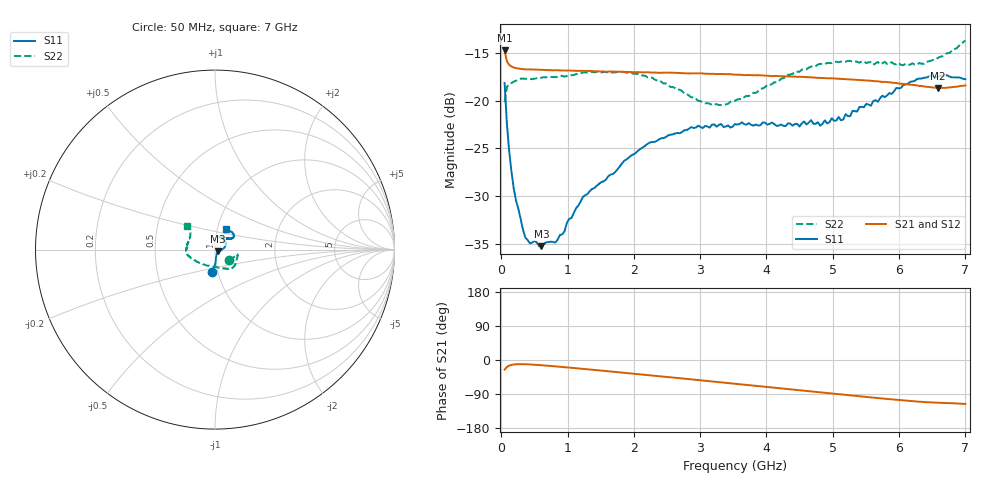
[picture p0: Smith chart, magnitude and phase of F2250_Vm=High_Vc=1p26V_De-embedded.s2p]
! Integrated Device Technology
! Corporate Headquarters
! 6024 Silver Creek Valley Road
! San Jose, CA 95138  USA
! Phone:  1-408-284-8200
! Toll Free:  1-800-223-1366
! Webpage:  http://www.idt.com/
! Timing and RF Division
! 515 Groton Road, Suite 102
! Westford, MA 01886-6024
! Device:  F2250
! Description: Voltage Variable RF Attenuator
! Frequency:  50.0 -  6000.00 MHz
! Package:  3x3 mm Thin QFN Plastic Package: 16 pin
! Ports:  2 RF, 3 DC
!  Pin  1  = GND
!  Pin  2  = NC
!  Pin  3  = RF1  = Port 1
!  Pin  4  = NC
!  Pin  5  = GND
!  Pin  6  = GND
!  Pin  7  = GND
!  Pin  8  = GND
!  Pin  9  = NC
!  Pin 10  = RF2  = Port 2
!  Pin 11  = NC
!  Pin 12  = GND
!  Pin 13  = GND
!  Pin 14  = VCNTRL
!  Pin 15  = VDD
!  Pin 16  = VMODE
! Vcntrl:  1.260 Volts
! Vmode:  +3.300 Volts
! Vdd:  +3.30  Volts
! Current:  1.331 mA
! Data:  The device was measured on a the F2250 evaluation board which has
!  individual transmission lines to the RF pins.  Data was collected
!  using a calibrated network analyzer.  The evaluation board was
!  de-embedded using a TRL calibration technique.
!  The reference plane is the edge of the package pin.
! Misc:  SN 10
!  Action Tracker AT0258
! Date Measured:  2014-11-26
! Date:  2015-10-15  MJV
! Note:
!  Integrated Device Technology supplies this data as a sample of measured
!  data at the package pin for this product.  Your particular data for this
!  product may vary.
!  Data was taken at 25 degrees C.
!  Integrated Device Technology reserves the right to change this data at anytime.
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# GHz S dB R 50
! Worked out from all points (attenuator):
!   201 points, 50 MHz to 7 GHz, reference 50 ohm
!   highest |S21| = -14.73 dB at 50 MHz (marker M1); lowest = -18.7 dB at 6.583 GHz (marker M2)
!   lowest |S11| = -35.3 dB at 606 MHz (marker M3), VSWR 1.04, Z = 51.5 - j0.891 ohm
!   |S11| at or under -10 dB: start of sweep to end of sweep
!   |S22| runs from -20.5 to -13.7 dB; largest |S21 - S12| = 0.00058
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0.05  -18.15 -96.5  -14.73 -25.5  -14.73 -25.4  -20.15 -38.1
0.08475  -22.44 -88.0  -15.87 -18.4  -15.86 -18.3  -18.56 -18.7
0.1195  -25.31 -85.2  -16.25 -14.8  -16.24 -14.7  -18.26 -13.5
0.189  -29.26 -77.5  -16.53 -11.8  -16.52 -11.8  -18.00 -11.9
0.22375  -30.51 -72.3  -16.59 -11.2  -16.58 -11.2  -17.90 -12.3
0.36275  -34.35 -54.9  -16.72 -11.1  -16.70 -11.1  -17.71 -13.3
0.606  -35.26 -30.1  -16.77 -13.8  -16.77 -13.8  -17.59 -19.8
0.8145  -34.88 -18.1  -16.81 -16.8  -16.80 -16.8  -17.52 -25.6
1.2315  -30.09 -9.1  -16.87 -23.4  -16.86 -23.4  -17.04 -35.8
1.96125  -25.74 11.6  -16.99 -35.6  -17.01 -35.6  -17.11 -48.8
2.37825  -24.07 22.6  -17.07 -42.6  -17.07 -42.7  -17.84 -57.5
3.07325  -22.65 44.4  -17.18 -54.7  -17.17 -54.8  -20.28 -87.3
3.525  -22.45 58.6  -17.27 -62.7  -17.26 -62.7  -20.00 -118.3
4.7065  -22.42 66.1  -17.57 -83.5  -17.58 -83.4  -16.45 -166.0
5.15825  -21.98 48.9  -17.73 -91.4  -17.74 -91.4  -15.87 -175.3
5.193  -21.41 49.1  -17.74 -92.0  -17.75 -92.0  -15.92 -176.2
5.2625  -21.62 45.7  -17.78 -93.2  -17.78 -93.2  -15.83 -177.2
5.29725  -21.05 44.9  -17.79 -93.8  -17.80 -93.9  -15.92 -178.1
5.85325  -19.21 34.6  -18.08 -103.3  -18.08 -103.4  -16.14 168.0
6.27025  -17.73 35.1  -18.40 -109.6  -18.40 -109.7  -16.22 154.8
6.583  -17.47 41.6  -18.67 -112.7  -18.65 -112.8  -15.52 144.1
7  -17.75 62.6  -18.41 -116.0  -18.40 -116.2  -13.68 139.7
